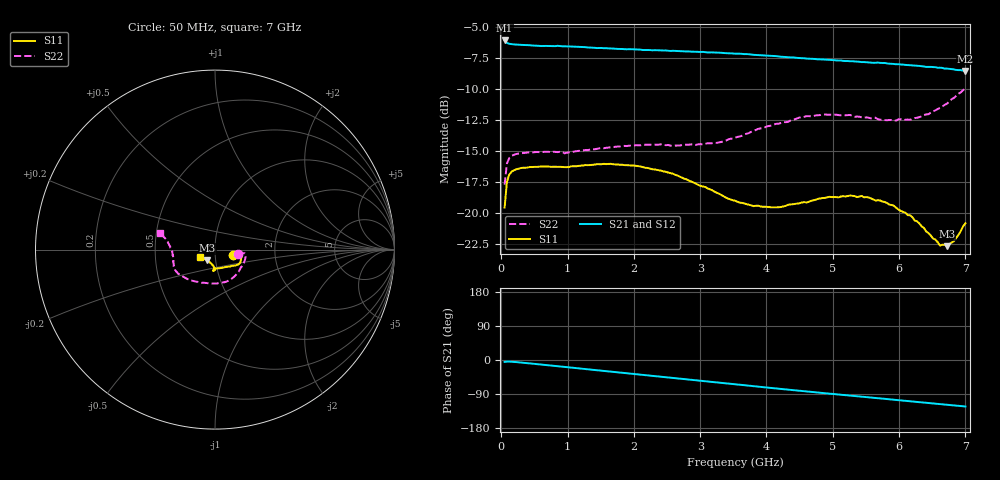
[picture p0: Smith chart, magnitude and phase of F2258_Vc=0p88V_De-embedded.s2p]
! Integrated Device Technology
! Corporate Headquarters
! 6024 Silver Creek Valley Road
! San Jose, CA 95138  USA
! Phone:  1-408-284-8200
! Toll Free:  1-800-223-1366
! Webpage:  http://www.idt.com/
! Timing and RF Division
! 515 Groton Road, Suite 102
! Westford, MA 01886-6024
! Device:  F2258
! Description: Voltage Variable RF Attenuator
! Frequency:  50.0 -  6000.00 MHz
! Package:  3x3 mm Thin QFN Plastic Package: 16 pin
! Ports:  2 RF, 2 DC
!  Pin  1  = NC
!  Pin  2  = NC
!  Pin  3  = RF2  = Port 2
!  Pin  4  = GND
!  Pin  5  = Vdd
!  Pin  6  = NC
!  Pin  7  = VCTRL
!  Pin  8  = NC
!  Pin  9  = GND
!  Pin 10  = RF1  = Port 1
!  Pin 11  = NC
!  Pin 12  = NC
!  Pin 13  = NC
!  Pin 14  = NC
!  Pin 15  = NC
!  Pin 16  = NC
! Vcntrl:  0.880 Volts
! Vdd:  +3.300 Volts
! Current:  1.145 mA
! Data:  The device was measured on a the F2258 evaluation board which has
!  individual transmission lines to the RF pins.  Data was collected
!  using a calibrated network analyzer.  The evaluation board was
!  de-embedded using a TRL calibration technique.
!  The reference plane is the edge of the package pin.
! Misc:  SN 10
!  Action Tracker AT0285
! Date Measured:  2014-12-10
! Date:  2016-01-13  MJV
! Note:
!  Integrated Device Technology supplies this data as a sample of measured
!  data at the package pin for this product.  Your particular data for this
!  product may vary.
!  Data was taken at 25 degrees C.
!  Integrated Device Technology reserves the right to change this data at anytime.
!Freq_(GHz)  S11M_(dB)  S11P_(deg)  S21M_(dB)  S21P_(deg)  S12M_(dB)  S12P_(deg)  S22M_(dB)  S22P_(deg)
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# GHz S dB R 50
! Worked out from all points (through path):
!   201 points, 50 MHz to 7 GHz, reference 50 ohm
!   highest |S21| = -6.10 dB at 50 MHz (marker M1); lowest = -8.6 dB at 7 GHz (marker M2)
!   group delay of S21, straight-line fit = 48.3 ps
!   lowest |S11| = -22.6 dB at 6.722 GHz (marker M3), VSWR 1.16, Z = 45.6 - j5.52 ohm
!   |S11| at or under -10 dB: start of sweep to end of sweep
!   |S22| runs from -17.7 to -9.9 dB; largest |S21 - S12| = 0.0026
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0.05  -19.53 -15.3  -6.10 -5.0  -6.09 -5.0  -17.68 -11.6
0.08475  -17.47 -7.9  -6.29 -4.2  -6.28 -4.2  -15.99 -7.2
0.1195  -16.89 -5.9  -6.36 -4.2  -6.34 -4.2  -15.55 -7.0
0.189  -16.54 -5.7  -6.42 -5.0  -6.40 -5.0  -15.29 -8.4
0.6755  -16.24 -13.5  -6.54 -13.3  -6.50 -13.3  -15.05 -23.6
0.9535  -16.28 -19.5  -6.56 -18.4  -6.57 -18.4  -15.17 -33.4
1.2315  -16.15 -23.3  -6.63 -23.3  -6.63 -23.3  -14.93 -42.1
1.6485  -16.01 -28.1  -6.74 -30.7  -6.73 -30.7  -14.68 -53.9
2.37825  -16.53 -35.0  -6.89 -43.4  -6.88 -43.4  -14.47 -73.8
3.0385  -17.83 -46.2  -7.01 -55.1  -7.03 -55.1  -14.45 -96.0
3.525  -18.98 -61.2  -7.16 -64.0  -7.15 -64.0  -13.92 -115.5
3.803  -19.42 -72.8  -7.25 -69.0  -7.25 -69.0  -13.36 -125.9
4.081  -19.52 -82.1  -7.34 -73.9  -7.34 -73.9  -12.93 -134.6
4.7065  -18.95 -94.5  -7.58 -84.7  -7.58 -84.7  -12.18 -149.2
4.94975  -18.66 -95.4  -7.65 -88.8  -7.65 -88.8  -12.07 -153.2
5.43625  -18.60 -92.9  -7.84 -96.8  -7.82 -96.8  -12.28 -161.1
5.85325  -19.30 -90.8  -7.97 -103.7  -7.95 -103.7  -12.49 -169.7
6.166  -20.15 -92.8  -8.08 -108.9  -8.07 -108.9  -12.48 -176.9
6.61775  -22.58 -115.1  -8.29 -116.5  -8.29 -116.5  -11.52 171.1
6.722  -22.64 -125.4  -8.36 -118.3  -8.35 -118.3  -11.19 168.3
6.82625  -22.24 -136.7  -8.42 -119.9  -8.44 -119.9  -10.72 166.4
7  -20.79 -155.0  -8.55 -122.7  -8.56 -122.7  -9.91 162.8
